ORGANIZATION_BLOCK MAIN:OB1
TITLE=

BEGIN
NETWORK 1
LD Q0.0
A I0.2
O I0.1
A I0.0
AN Q0.3
A I0.5
= S0.0

NETWORK 2
LSCR S0.0

NETWORK 3
LD I0.0
= Q0.0

NETWORK 4
LD Q0.1
ON Q0.2
TON T32 +50

NETWORK 5
LDN T32
AN Q0.2
= Q0.1

NETWORK 6
LD T32
O Q0.2
AN Q0.1
= Q0.2

NETWORK 7
SCRE

NETWORK 8
LD Q0.2
ED
LD T33
CTU C0 +4

NETWORK 9
LD Q0.3
A I0.4
O I0.3
O C0
AN T33
A I0.5
= Q0.3

NETWORK 10
LD Q0.3
TON T33 +100

NETWORK 11
LDN Q0.0
= Q0.4

NETWORK 12
LD Q0.1
O Q0.2
= Q0.5

NETWORK 13
LDN Q0.3
= Q0.6

NETWORK 14
LD Q0.3
= Q0.7

END_ORGANIZATION_BLOCK

